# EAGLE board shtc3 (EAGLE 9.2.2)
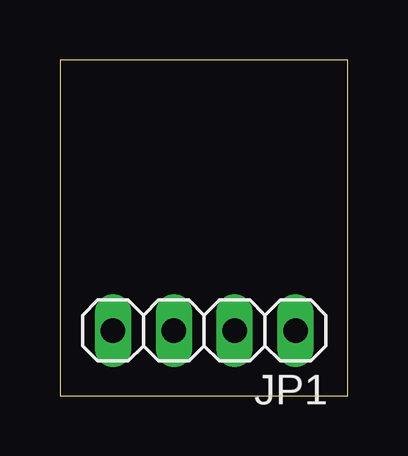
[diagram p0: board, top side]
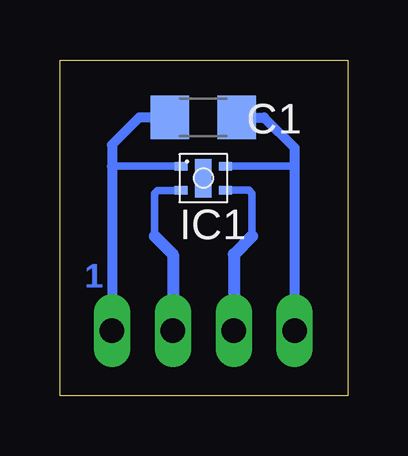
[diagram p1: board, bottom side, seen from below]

Size 12 x 14.02 mm. Coordinates in mm from the lower left corner, seen from the top.
Outline: 0,0.01 12,0 12,14.02 0,14.01 0,0.01
Copper layers (1*16): Top 0.035mm / dielectric 1.5mm / Bottom 0.035mm
Design rules "default": minimum track width 6mil, minimum drill 0.35mm, track to track 6mil, track to pad 6mil, pad to pad 6mil, via to via 6mil, smd to smd 6mil, copper to edge 40mil, drill to drill 6mil, minimum pad ring 10mil, minimum via ring 8mil, stop-mask expansion 4mil, vias tented up to drill 0mil, thermal gap 10mil

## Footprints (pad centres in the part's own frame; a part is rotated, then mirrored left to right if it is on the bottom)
C1206 = smd 1.6 x 1.8: 1 -1.4,0; 2 1.4,0
DFN4 = smd 0.7 x 1.6: 0 0,0 | smd 0.55 x 0.35: 1 -0.925,0.5; 2 -0.925,-0.5; 3 0.925,-0.5; 4 0.925,0.5
1X04 = drill 1.016 long: 1 -3.81,0; 2 -1.27,0; 3 1.27,0; 4 3.81,0

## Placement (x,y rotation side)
C1  100n  [C1206]  6.02,11.62 180 bottom
IC1  SHTC3  [DFN4]  6.02,9.08 0 bottom
JP1  [1X04]  6.02,2.73 180 top

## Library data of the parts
C1 = rcl
IC1 = #Matej
JP1 = pinhead

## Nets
SCL: IC1.2 JP1.2
SDA: IC1.3 JP1.3
VDD: C1.2 IC1.1 JP1.1
VSS: C1.1 IC1.4 JP1.4

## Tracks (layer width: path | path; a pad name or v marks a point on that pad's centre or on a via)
SCL
  Bottom 0.305: IC1.2 6.95,8.57 7.92,8.57 8.05,8.45 8.05,6.67
  Bottom 0.508: 8.05,6.67 7.29,5.9 JP1.2
SDA
  Bottom 0.305: IC1.3 4.12,8.58 3.99,8.45 3.99,6.67
  Bottom 0.508: 3.99,6.67 4.75,5.9 JP1.3
VDD
  Bottom 0.305: IC1.1 9.82,9.58 9.83,9.59
  Bottom 0.406: C1.2 8.69,11.62 9.83,10.48 9.83,9.59 JP1.1
VSS
  Bottom 0.305: IC1.4 2.22,9.58 2.21,9.59
  Bottom 0.406: C1.1 3.48,11.62 2.21,10.35 2.21,9.59 JP1.4

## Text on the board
Bottom: 1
